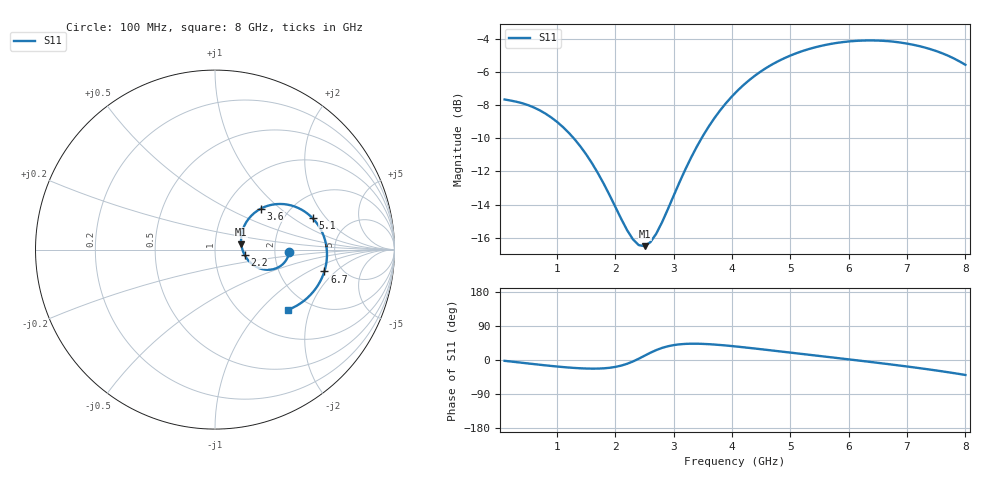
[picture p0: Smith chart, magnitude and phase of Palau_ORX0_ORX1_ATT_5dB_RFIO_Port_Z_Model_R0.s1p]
! Created Fri Jul 10 10:30:47 2020
! Palau ORX0/ORX1 RFIO Port Impedance Model.
! Attenuation : 5 dB.
! Revision		: R0.
! Impedance Mode 	: Balanced Differential-Mode.
! Impedance Format 	: Series Equivalent Differential Impedance (SEDZ).
# hz S ma R 50
! 1 Port Network Data from SP1.SP block
! freq  magS11  angS11
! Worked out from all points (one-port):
!   80 points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, 100 MHz to 8 GHz, reference 50 ohm
!   lowest |S11| = -16.5 dB at 2.5 GHz (marker M1), VSWR 1.35, Z = 67 + j4.03 ohm
!   |S11| at or under -10 dB: 1.287 GHz to 3.476 GHz (2.189 GHz wide, 91.9 % of centre)
!   S11 on the Smith chart (normalised r, x): 100 MHz: 2.41, -0.09; 2.2 GHz: 1.39, -0.08; 3.6 GHz: 1.46, +0.76; 5.1 GHz: 2.83, +1.47; 6.7 GHz: 3.67, -1.46; 8 GHz: 1.55, -1.45
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1e8  0.4146 -2.2
6e8  0.3923 -10.8
1.1e9  0.3423 -18.6
1.4e9  0.299 -21.9
1.6e9  0.2657 -22.8
1.8e9  0.2306 -22.0
2.1e9  0.1805 -14.8
2.2e9  0.167 -10.0
2.3e9  0.1567 -3.9
2.4e9  0.1505 3.4
2.5e9  0.1494 11.4
2.6e9  0.1537 19.2
2.7e9  0.163 26.2
3.1e9  0.2334 41.4
3.4e9  0.2996 43.0
3.6e9  0.3436 41.7
3.8e9  0.3853 39.5
4.1e9  0.442 35.1
4.3e9  0.4753 31.8
4.6e9  0.5182 26.6
5.1e9  0.5719 17.7
5.6e9  0.6059 8.8
6.1e9  0.6228 -0.1
6.4e9  0.6251 -5.6
6.7e9  0.6215 -11.3
7.1e9  0.6069 -19.2
7.6e9  0.572 -29.9
8e9  0.5278 -39.5
